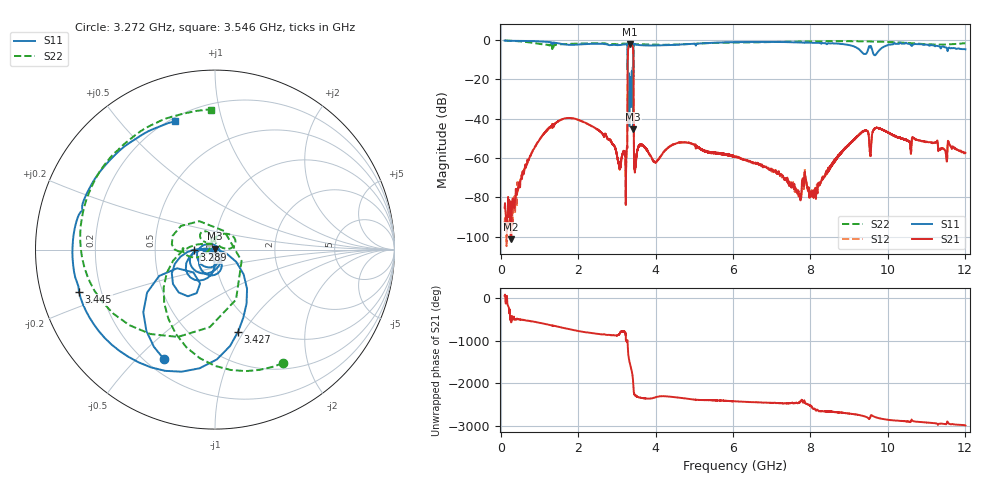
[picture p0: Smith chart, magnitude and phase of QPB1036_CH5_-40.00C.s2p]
! TDS: K:\Engsetup\Winsaw\QPB1036_ALL
! Channel 1
! Ports=1 2
! seg 1=100.000000 1100.000000 101
! seg 2=1101.000000 1501.000000 401
! seg 3=1502.000000 2502.000000 101
! seg 4=2503.000000 3803.000000 1301
! seg 5=3804.000000 5004.000000 121
! seg 6=5005.000000 6005.000000 1001
! seg 7=6006.000000 8406.000000 241
! seg 8=8407.000000 10607.000000 2201
! seg 9=10608.000000 12008.000000 141
! Points=5609
! FailCode=0
! Topology=ALL_SE(12)
!VNA Cal loaded =QPB1036_ALL_-40C
!PS1(V)= 5.000
!PS(mA)= 0.500
!PS2(V)= 1.170
!PS(mA)= -0.100
!PS3(V)= 0.630
!PS(mA)= 0.100
!PS4(V)= 1.170
!PS(mA)= -0.100
!Temp (C)= -40.00
# MHz S DB R 50
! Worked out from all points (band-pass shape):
!   5609 points, 100 MHz to 12.01 GHz, reference 50 ohm
!   highest |S21| = -2.27 dB at 3.344 GHz (marker M1); lowest = -101.3 dB at 270 MHz (marker M2)
!   |S21| within 3 dB of the highest: 3.29 GHz to 3.423 GHz (132.9 MHz wide, 3.96 % of centre)
!   lowest |S11| = -45.5 dB at 3.42 GHz (marker M3), VSWR 1.01, Z = 49.8 + j0.486 ohm
!   |S11| at or under -10 dB: 3.277 GHz to 3.425 GHz (147.3 MHz wide, 4.4 % of centre)
!   |S22| runs from -30.8 to -0.3 dB; largest |S21 - S12| = 0.0077
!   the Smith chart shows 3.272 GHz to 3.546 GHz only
!   S11 on the Smith chart (normalised r, x): 3.272 GHz: 0.27, -0.60; 3.289 GHz: 0.79, -0.00; 3.427 GHz: 0.80, -0.94; 3.445 GHz: 0.12, -0.15; 3.546 GHz: 0.22, +0.71
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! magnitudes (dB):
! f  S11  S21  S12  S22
! 100 MHz  -0.3  -85.3  -93.8  -0.3
! 270 MHz  -0.4  -101.3  -82.7  -0.4
! 1.205 GHz  -1.0  -45.6  -45.8  -2.4
! 2.092 GHz  -2.2  -41.3  -41.3  -1.8
! 3.075 GHz  -2.6  -65.4  -65.3  -2.1
! 3.242 GHz  -2.1  -62.8  -62.9  -1.9
! 3.272 GHz  -3.4  -44.8  -44.8  -2.6
! 3.289 GHz  -18.5  -5.5  -5.5  -22.4
! 3.344 GHz  -19.0  -2.3  -2.3  -25.3
! 3.401 GHz  -27.8  -2.8  -2.8  -26.7
! 3.42 GHz  -45.5  -4.4  -4.4  -14.6
! 3.427 GHz  -6.5  -8.9  -8.9  -18.7
! 3.445 GHz  -2.0  -65.0  -64.6  -2.3
! 3.469 GHz  -2.1  -65.0  -66.3  -2.2
! 3.546 GHz  -2.5  -54.9  -55.3  -2.1
! 4.074 GHz  -2.8  -60.5  -60.9  -2.4
! 6.056 GHz  -1.1  -59.1  -59.1  -1.3
! 8.046 GHz  -1.4  -79.6  -79.8  -0.7
! 9.349 GHz  -6.5  -46.5  -46.5  -0.7
! 9.549 GHz  -3.7  -58.0  -58.3  -0.8
! 10.02 GHz  -2.3  -47.1  -47.2  -1.1
! 12.01 GHz  -4.8  -57.4  -57.5  -1.7
